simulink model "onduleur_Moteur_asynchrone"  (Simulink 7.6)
settings: Solver=FixedStepDiscrete  StartTime=0.0  StopTime=N  FixedStep=Ts  RelTol=1e-3
InitFcn:
  | clc
  | close all
  | clear all
  | Ts=1e-5;
  | N=100;
undefined symbols (not defined in the file or in its folder): arm, bridge, pulses
libraries: powerlib x6, powerlib_extras x1

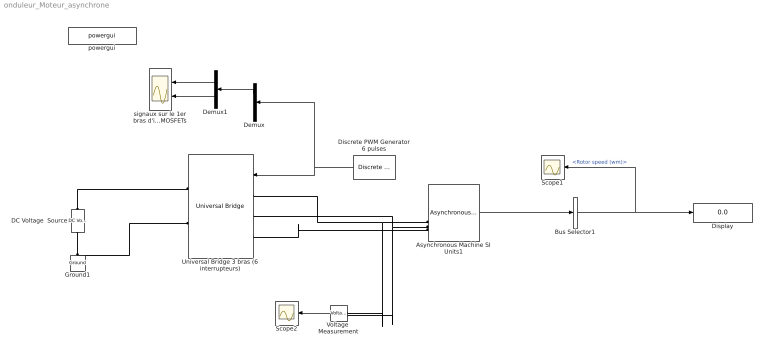
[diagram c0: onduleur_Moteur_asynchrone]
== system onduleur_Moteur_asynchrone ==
  Asynchronous Machine SI Units1 : powerlib/Machines/Asynchronous Machine SI Units  DialogController=POWERSYS.PowerSysDialog  SystemSampleTime=-1  PresetModel=No  MechanicalLoad=Torque Tm  ShowDetailedParameters=on  RotorType=Squirrel-cage  ReferenceFrame=Stationary  NominalParameters=[ 3800, 380, 60 ]  Stator=[ 0.029 1e-4]  Rotor=[ 0.022 1e-4]  Cage1=[ 0.022 0.226/377]  Cage2=[ 0.022 0.226/377]  Lm=0.05  Mechanical="[50 0  2 ]"  PolePairs=2  InitialConditions=[1 0 0 0 0 0 0 0]  Units=SI  LoadFlowParameters=1492000  SimulateSaturation=off  Saturation=[14.03593122, 27.81365428, 53.79336849, 72.68890987, 97.98006896, 148.6815601, 215.7428561, 302.9841135, 428.7778367 ; 230, 322, 414, 460, 506, 552, 598, 644, 690]  TsPowergui=0  TsBlock=-1  IterativeModel=Forward Euler
  Bus Selector1 : BusSelector  OutputSignals=Mechanical.Rotor speed (wm)
  DC Voltage  Source : powerlib/Electrical Sources/DC Voltage Source  DialogController=POWERSYS.PowerSysDialog  SystemSampleTime=-1  Amplitude=380  Measurements=None
  Demux : Demux  Outputs=3
  Demux1 : Demux  Outputs=2
  Discrete PWM Generator 6 pulses : powerlib_extras/Discrete  Control Blocks/Discrete PWM Generator  DialogController=POWERSYS.PowerSysDialog  SystemSampleTime=-1  GeneratorMode="3-arm  bridge (6 pulses)"  Fc=1080  Ts=Ts  Internal=on  mIndex=0.8  Freq=60  Phase=0
  Display : Display
  Ground1 : powerlib/Elements/Ground  DialogController=POWERSYS.PowerSysDialog  PhysicalDomain=powersysdomain  SubClassName=unknown  LeftPortType=p1  RightPortType=p1  LConnTagsString=a
  Scope1 : Scope
  Scope2 : Scope
  Universal Bridge 3 bras (6 interrupteurs) : powerlib/Power Electronics/Universal Bridge  DialogController=POWERSYS.PowerSysDialog  SystemSampleTime=-1  Arms=3  SnubberResistance=1e5  SnubberCapacitance=inf  Device=MOSFET / Diodes  Ron=1e-4  Lon=0  ForwardVoltages="[  1  1  ]"  ForwardVoltage=.8  GTOparameters=[ 10e-6 , 20e-6 ]  IGBTparameters=[ 1e-6 , 2e-6 ]  Measurements=None  Measurements_2=None  converterType=Rectifier
  Voltage  Measurement : powerlib/Measurements/Voltage Measurement  DialogController=POWERSYS.PowerSysDialog  SystemSampleTime=-1  PhasorSimulation=off  OutputType=Complex  PSBequivalent=0
  powergui : powerlib/powergui  Priority=2  SystemSampleTime=-1  SimulationMode=Discrete  SampleTime=Ts  frequency=60  SPID=off  DisableSnubberDevices=off  DisableRonSwitches=off  DisableVfSwitches=off  SwTol=0  Interpol=off  frequencyindice=0  echomessages=off  HookPort=off  DisplayEquations=off  FunctionMessages=off  EnableUseOfTLC=off  x0status=blocks  RestoreLinks=warning  ResistiveCurrentMeasurement=off  Frange=[0:2:500]  Ylog=off  Xlog=off  ShowGrid=off  save=off  variable=ZData  structure=psb3phPWM1_str  ZoomFFT=on  StartTime=0.1 - 2/60  cycles=2  DisplayStyle=off  fundamental=60  FreqAxis=off  MaxFrequency=5000  frequencyindicesteady=1  RmsSteady=1  display=off  Ts=0  methode=off
  signaux sur le 1er bras d'interrupteurs MOSFETs : Scope  NumInputPorts=2
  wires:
  Discrete PWM Generator 6 pulses/1 -> Universal Bridge 3 bras (6 interrupteurs)/1, Demux/1
  Asynchronous Machine SI Units1/1 -> Bus Selector1/1
  Bus Selector1/1 -> Display/1, Scope1/1  "<Rotor speed (wm)>"
  Voltage  Measurement/1 -> Scope2/1
  Demux/1 -> Demux1/1
  Demux1/1 -> signaux sur le 1er bras d'interrupteurs MOSFETs/1
  Demux1/2 -> signaux sur le 1er bras d'interrupteurs MOSFETs/2
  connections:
  Ground1/LConn1 -- Universal Bridge 3 bras (6 interrupteurs)/RConn2 -- DC Voltage  Source/LConn1
  DC Voltage  Source/RConn1 -- Universal Bridge 3 bras (6 interrupteurs)/RConn1
  Asynchronous Machine SI Units1/LConn1 -- Universal Bridge 3 bras (6 interrupteurs)/LConn1 -- Voltage  Measurement/LConn1
  Universal Bridge 3 bras (6 interrupteurs)/LConn3 -- Asynchronous Machine SI Units1/LConn3
  Asynchronous Machine SI Units1/LConn2 -- Universal Bridge 3 bras (6 interrupteurs)/LConn2 -- Voltage  Measurement/LConn2
